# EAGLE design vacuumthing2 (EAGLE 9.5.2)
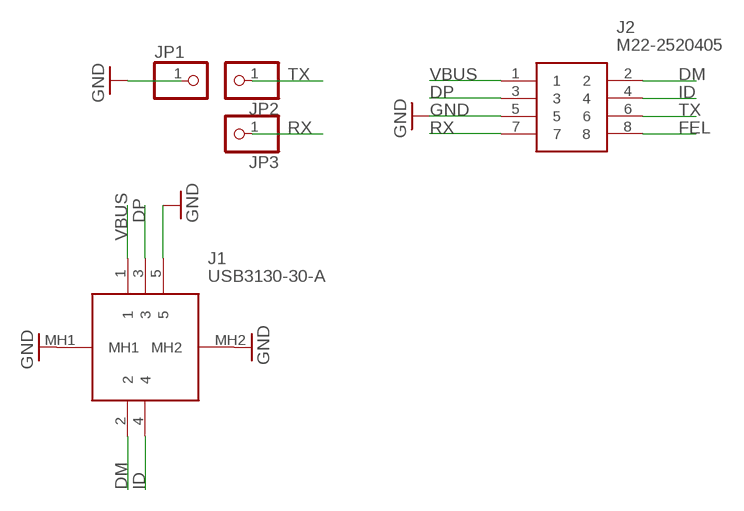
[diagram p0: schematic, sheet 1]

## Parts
J1  USB3130-30-A  [USB313030A]
J2  M22-2520405  [HDRV8W60P200_2X4_800X400X500P]
JP1  PINHD-1X1  [1X01]
JP2  PINHD-1X1  [1X01]
JP3  PINHD-1X1  [1X01]

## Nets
DM: J1.2 J2.2
DP: J1.3 J2.3
FEL: J2.8
GND: J1.5 J1.MH1 J1.MH2 J2.5 JP1.1
ID: J1.4 J2.4
RX: J2.7 JP3.1
TX: J2.6 JP2.1
VBUS: J1.1 J2.1

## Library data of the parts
J1 = SamacSys_Parts:USB3130-30-A: GCT (GLOBAL CONNECTOR TECHNOLOGY) - USB3130-30-A - USB Connector, Micro USB Type B, USB 2.0, Receptacle, 5 Ways, Through Hole Mount, Vertical Source: Datasheet; DESCRIPTION: GCT (GLOBAL CONNECTOR TECHNOLOGY) - USB3130-30-A - USB Connector, Micro USB Type B, USB 2.0, Receptacle, 5 Ways, Through Hole Mount, Vertical; HEIGHT: 5.6mm; MANUFACTURER_NAME: GCT (GLOBAL CONNECTOR TECHNOLOGY); MANUFACTURER_PART_NUMBER: USB3130-30-A
J2 = SamacSys_Parts:M22-2520405: HARWIN - M22-2520405 - CONNECTOR, HEADER, 8POS, 2ROW, 2MM Source: Datasheet; DESCRIPTION: HARWIN - M22-2520405 - CONNECTOR, HEADER, 8POS, 2ROW, 2MM; HEIGHT: 5mm; MANUFACTURER_NAME: Harwin; MANUFACTURER_PART_NUMBER: M22-2520405; MOUSER_PART_NUMBER: 855-M22-2520405; MOUSER_PRICE-STOCK: https://www.mouser.com/Search/Refine.aspx?Keyword=855-M22-2520405
JP1-JP3 = pinhead:PINHD-1X1: PIN HEADER

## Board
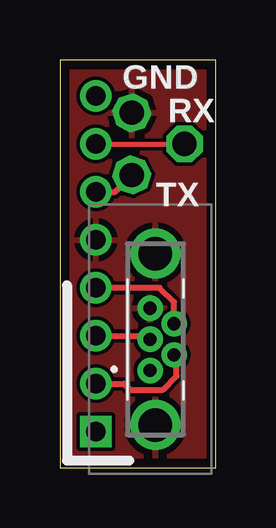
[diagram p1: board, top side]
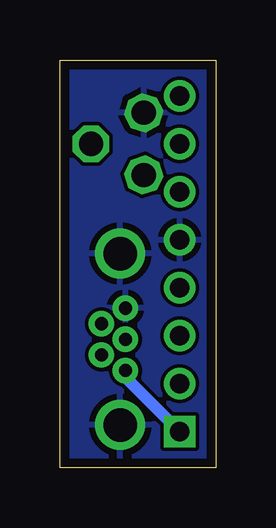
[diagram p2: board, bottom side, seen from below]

Size 6.5 x 17 mm. Coordinates in mm from the lower left corner, seen from the top.
Outline: 0,0 6.5,0 6.5,17 0,17 0,0
Copper layers (1*16): Top 0.035mm / dielectric 1.5mm / Bottom 0.035mm
Design rules "default *": minimum track width 6mil, minimum drill 0.35mm, track to track 6mil, track to pad 6mil, pad to pad 6mil, via to via 6mil, smd to smd 6mil, copper to edge 15mil, drill to drill 6mil, minimum pad ring 10mil, minimum via ring 0.13mm, stop-mask expansion 0mil, vias tented up to drill 30mil, thermal gap 10mil

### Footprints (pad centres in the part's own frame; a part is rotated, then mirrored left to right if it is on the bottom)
USB313030A = drill 0.55 pad 1: 1 0,0; 2 0.65,-1; 3 1.3,0; 4 1.95,-1; 5 2.6,0 | drill 1.39 pad 2.085: MH1 -2.275,-0.22; MH2 4.875,-0.22
HDRV8W60P200_2X4_800X400X500P = drill 0.8 pad 1.2 square: 1 0,0 | drill 0.8 pad 1.2: 2 -2,0; 3 -4,0; 4 -6,0; 5 -8,0; 6 -10,0; 7 -12,0; 8 -14,0
1X01 = drill 1.016 octagon: 1 0,0

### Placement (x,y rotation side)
J1  3.76,4.05 90 top
J2  1.5,1.5 270 bottom
JP1  3,14.8 17 top
JP2  3,12.2 27 top
JP3  5.2,13.5 90 top

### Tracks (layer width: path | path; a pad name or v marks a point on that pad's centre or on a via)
DM
  Top 0.254: J2.2 2.67,3.5 2.93,3.24 4.3,3.24 4.87,3.81 4.87,4.59 J1.2
DP
  Top 0.254: J2.3 3.61,5.5 J1.3
GND
  pour Bottom: -0.77,20.32 -0.77,-1.27 10.66,-1.27 10.66,20.32
  pour Top: -0.77,20.32 -0.77,-1.27 10.66,-1.27 10.66,20.32
ID
  Top 0.254: J1.4 4.76,6.9 4.16,7.5 J2.4
RX
  Top 0.2: J2.7 JP3.1
TX
  Top 0.254: J2.6 2.3,11.5 JP2.1
VBUS
  Bottom 0.508: J2.1 3.76,3.76 J1.1

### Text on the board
tNames: GND | RX | TX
